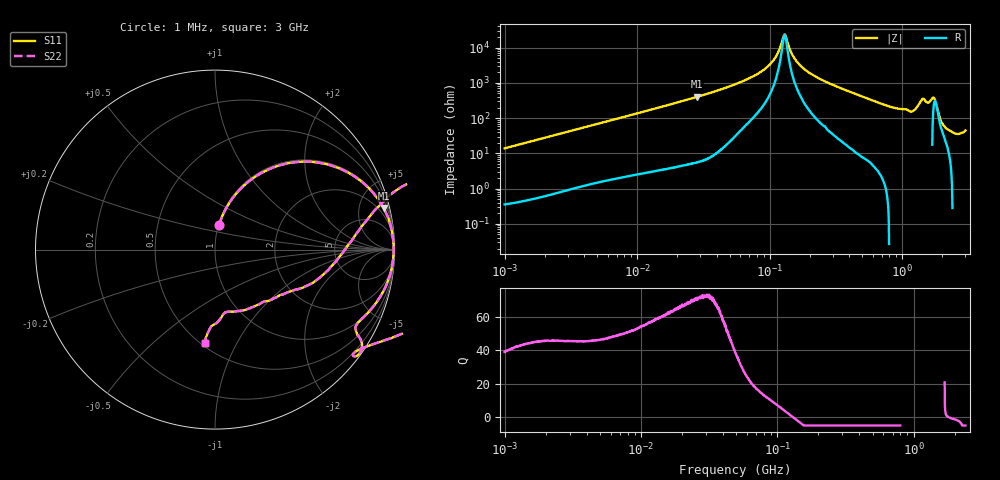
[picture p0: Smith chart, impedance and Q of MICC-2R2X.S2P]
!s-Parameter Generated by FASTRON Sdn. Bhd.
!FASTRON P/N : MICC-2R2X
!Keysight Technologies,E4991B,MY54100416,A.01.15
!Date: Fri Aug 28 09:31:39 2026
!Version  : Rev00 Fri Aug 28 09:31:39 2026
!Data & Calibration Information:
!PortZ  Port1:50+j0  Port2:50+j0
!When reading, reference impedance value at option line is always used.
!Remarks : This data is being provided solely for informational purposes.
!Freq	S11	S21	S12	S22
# Hz S dB R 50
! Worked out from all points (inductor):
!   1601 points, 1 MHz to 3 GHz, reference 50 ohm
!   read as one part in series: L = 2.21 uH near 1.041 MHz
!   highest Q = 72.3 at 28.44 MHz (marker M1), where L = 2.25 uH
!   self-resonance near 129.5 MHz
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1000000  -17.26 80.7  -0.11 -7.9  -0.11 -7.9  -17.26 80.7
3804036  -6.77 61.4  -1.12 -27.3  -1.12 -27.3  -6.77 61.4
7437954  -3.04 44.1  -3.15 -44.8  -3.15 -44.8  -3.04 44.1
1.447069e7  -1.05 26.7  -6.96 -62.4  -6.96 -62.4  -1.05 26.7
2.843618e7  -0.29 13.9  -12.38 -75.3  -12.38 -75.3  -0.29 13.9
5.477226e7  -0.08 6.3  -19.24 -81.8  -19.24 -81.8  -0.08 6.3
9.787053e7  -0.04 1.9  -29.65 -80.7  -29.65 -80.7  -0.04 1.9
1.125904e8  -0.04 0.9  -35.42 -74.8  -35.42 -74.8  -0.04 0.9
1.295243e8  -0.04 0.0  -47.32 -3.5  -47.32 -3.5  -0.04 0.0
1.574367e8  -0.04 -1.3  -32.86 77.7  -32.86 77.7  -0.04 -1.3
2.083556e8  -0.05 -3.3  -24.81 82.3  -24.81 82.3  -0.05 -3.3
7.925923e8  -0.84 -24.8  -7.54 65.1  -7.54 65.1  -0.84 -24.8
1.142072e9  -0.15 -37.2  -3.98 69.9  -3.98 69.9  -0.15 -37.2
1.243477e9  -0.09 -33.6  -4.80 72.2  -4.80 72.2  -0.09 -33.6
1.367504e9  1.72 -19.4  -7.30 110.2  -7.30 110.2  1.72 -19.4
1.488926e9  3.17 6.9  -6.68 -158.2  -6.68 -158.2  3.17 6.9
1.589003e9  1.99 18.9  -6.95 -114.9  -6.95 -114.9  1.99 18.9
1.747494e9  -1.77 8.1  -12.99 -30.7  -12.99 -30.7  -1.77 8.1
1.883708e9  -4.42 -15.4  -6.94 20.8  -6.94 20.8  -4.42 -15.4
2.020405e9  -6.87 -33.4  -3.48 21.9  -3.48 21.9  -6.87 -33.4
2.581816e9  -9.04 -79.1  -0.04 20.4  -0.04 20.4  -9.04 -79.1
3e9  -5.58 -96.3  1.43 26.3  1.43 26.3  -5.58 -96.3
